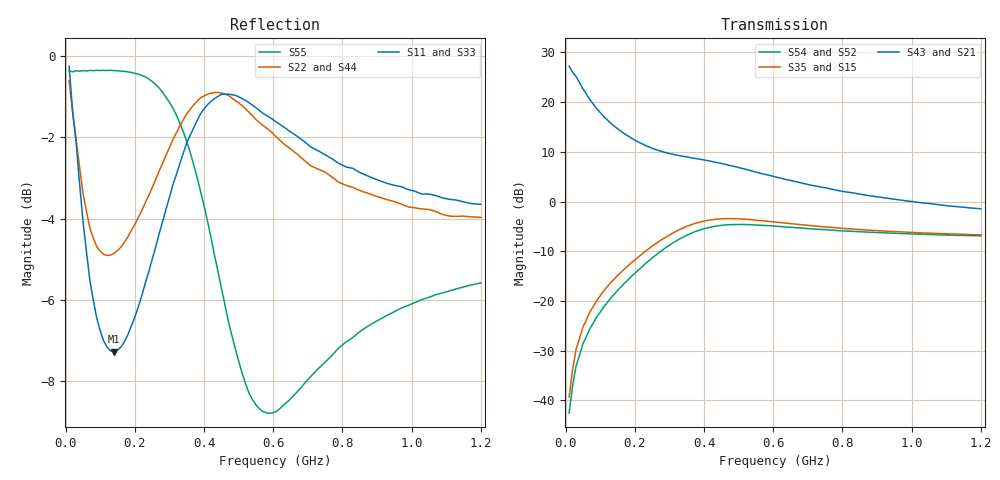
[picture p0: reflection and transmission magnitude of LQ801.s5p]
!  1/8/97
!  POLYFET RF DEVICES
!  LQ801
!  S PARAMETERS
!  VDS=28V, IDQ=200mA
! Date: Wed Jan 08 11:32:39 1997
! SCATTERING PARAMETERS :
!AWR Design Environment (2053) Wed Feb 04 15:25:28 2004
!freq-unit  param-type  data-format  keyword  impedance-ohms
# MHz  S  MA  R  50
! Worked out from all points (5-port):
!   120 points, 10 MHz to 1.2 GHz, reference 50 ohm
!   strongest paths, dB at 10 MHz, 310 MHz, 610 MHz, 910 MHz, 1.2 GHz:
!     S43: 27.2, 9.5, 4.9, 0.9, -1.5
!     S21: 27.2, 9.5, 4.9, 0.9, -1.5
!     S35: -39.3, -6.3, -4.1, -5.9, -6.7
!     S15: -39.3, -6.3, -4.1, -5.9, -6.7
!     S54: -42.6, -8.3, -5.0, -6.3, -6.9
!     S52: -42.6, -8.3, -5.0, -6.3, -6.9
!   lowest |S11| = -7.3 dB at 140 MHz (marker M1), VSWR 2.53, Z = 45.8 - j45.8 ohm
!   |S11| at or under -10 dB: nowhere
